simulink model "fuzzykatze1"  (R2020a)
settings: Solver=ode45  StartTime=0.0  StopTime=200  RelTol=1e-3  EnableMultiTasking=on
libraries: libregler2 x5

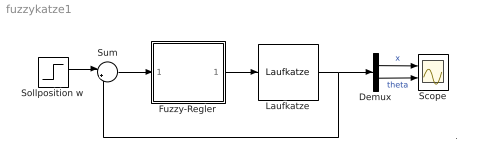
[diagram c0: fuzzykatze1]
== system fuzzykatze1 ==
  note: .
  Demux : Demux  Outputs=2
  Fuzzy-Regler : Subsystem  mask(Fuzzy Controller){bx=1, bth=0.001, Kp=20}
      mask prompts: bx "Breite Position"; bth "Breite Seilwinkel"; Kp "Regelverstaerkung"
  Laufkatze : libregler2/Laufkatze  mk=100  ml=500  l=3  g=9.81
  Scope : Scope  NumInputPorts=2
  Sollposition w : Step  Time=5  Before=[0,0]  After=[10,0]  SampleTime=0
  Sum : Sum  Inputs=|+-  SaturateOnIntegerOverflow=on
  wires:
  Fuzzy-Regler/1(u) -> Laufkatze/1
  Demux/1 -> Scope/1  "x"
  Demux/2 -> Scope/2  "theta"
  Laufkatze/1 -> Demux/1, Sum/2
  Sollposition w/1 -> Sum/1
  Sum/1 -> Fuzzy-Regler/1(e)

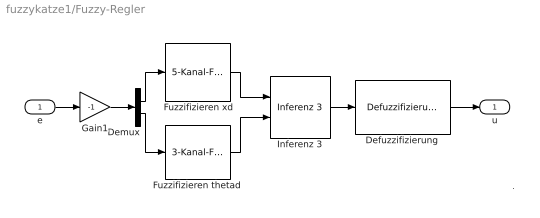
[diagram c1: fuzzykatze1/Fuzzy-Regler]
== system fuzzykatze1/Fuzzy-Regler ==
  note: .
  e : Inport
  " Fuzzifizieren xd" : libregler2/5-Kanal-Fuzzifizierer  w=bx  offset=0
  Defuzzifizierung : libregler2/Defuzzifizierung  h=[-1, 0, 1]*Kp
  Demux : Demux  Outputs=2
  Fuzzifizieren thetad : libregler2/3-Kanal-Fuzzifizierer  w=bth  offset=0
  Gain1 : Gain  Gain=-1  SaturateOnIntegerOverflow=on
  Inferenz 3 : libregler2/Inferenz 3  M=[3 3 3; 2 3 3; 1 2 3; 1 1 2; 1 1 1]
  u : Outport
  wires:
  e/1 -> Gain1/1
  Inferenz 3/1 -> Defuzzifizierung/1
  Defuzzifizierung/1 -> u/1
  Gain1/1 -> Demux/1
  Demux/1 -> " Fuzzifizieren xd"/1
  Demux/2 -> Fuzzifizieren thetad/1
  " Fuzzifizieren xd"/1 -> Inferenz 3/1
  Fuzzifizieren thetad/1 -> Inferenz 3/2
